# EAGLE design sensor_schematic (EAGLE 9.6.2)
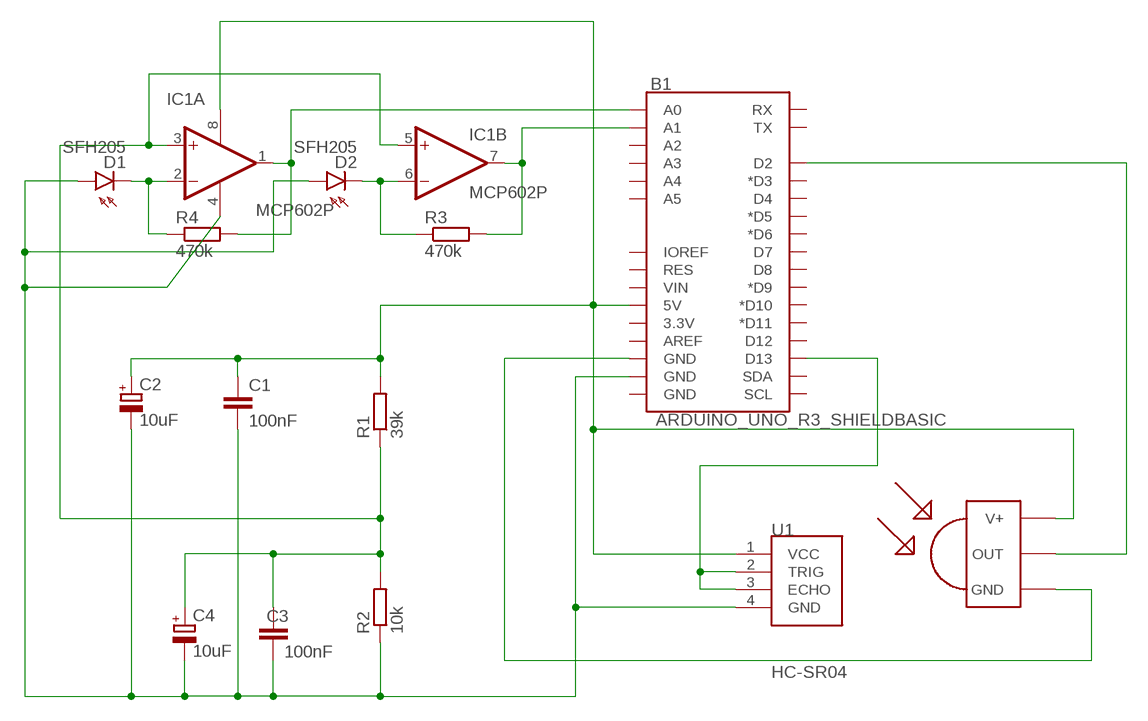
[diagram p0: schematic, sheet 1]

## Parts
B1  ARDUINO_UNO_R3_SHIELDBASIC  [UNO_R3_SHIELD]
C1  100nF  C-EU025-025X050  [C025-025X050]
C2  10uF  CPOL-EUE2.5-6  [E2,5-6]
C3  100nF  C-EU025-025X050  [C025-025X050]
C4  10uF  CPOL-EUE2.5-6  [E2,5-6]
D1  SFH205  [SFH205]
D2  SFH205  [SFH205]
IC1  MCP602P  [DIL08]
R1  39k  R-EU_0207/10  [0207/10]
R2  10k  R-EU_0207/10  [0207/10]
R3  470k  R-EU_0207/10  [0207/10]
R4  470k  R-EU_0207/10  [0207/10]
U1  HC-SR04  [XCVR_HC-SR04]
U$1  TSOP4856  [TSOP18XX]

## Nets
N$2: C3.1 C4.+ IC1.3(A:+IN) IC1.5(B:+IN) R1.1 R2.2
N$3: B1.5V C1.1 C2.+ IC1.8(P:V+) R1.2 U1.1(VCC) U$1.VCC(V+)
N$4: D2.K(C) IC1.6(B:-IN) R3.1
N$5: D1.K(C) IC1.2(A:-IN) R4.1
N$7: B1.GND@1(GND) C1.2 C2.- C3.2 C4.- D1.A D2.A IC1.4(P:V-) R2.1 U1.4(GND)
N$8: B1.GND@2(GND) U$1.GND
N$9: B1.D13 U1.2(TRIG) U1.3(ECHO)
N$10: B1.D2 U$1.OUT
N$11: B1.A0 IC1.1(A:OUT) R4.2
N$12: B1.A1 IC1.7(B:OUT) R3.2
Unconnected: B1.3.3V B1.A2 B1.A3 B1.A4 B1.A5 B1.AREF B1.D3(*D3) B1.D4 B1.D5(*D5) B1.D6(*D6) B1.D7 B1.D8 B1.D9(*D9) B1.D10(*D10) B1.D11(*D11) B1.D12 B1.GND@0(GND) B1.IOREF B1.RES B1.RX B1.SCL B1.SDA B1.TX B1.VIN

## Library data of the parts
B1 = SparkFun-Boards:ARDUINO_UNO_R3_SHIELD: Arduino R3 Shield Footprint Shield form compatible with the Arduino Uno R3. SparkFun Products: MG2639 Cellular Shield MIDI Shield R3 Stackable Headers Kit
C1 C3 = rcl:C-EU: CAPACITOR, European symbol; SPICEPREFIX: C
C2 C4 = rcl:CPOL-EU: POLARIZED CAPACITOR, European symbol; SPICEPREFIX: C
D1 D2 = opto-trans-siemens:SFH205: PHOTO DIODE; OC_FARNELL: unknown; OC_NEWARK: unknown
IC1 = linear:MCP602: Single Op Amp 2.7V to 6.0V Single Supply CMOS Source: http://ww1.microchip.com/downloads/en/DeviceDoc/21314g.pdf
R1-R4 = rcl:R-EU_: RESISTOR, European symbol; SPICEPREFIX: R
U1 = HC-SR04:HC-SR04: Ultrasonic Sensor Module Check availability; AVAILABILITY: Not in stock; DESCRIPTION: HC-SR04 Ultrasonic Sensor Qwiic Platform Evaluation Expansion Board; MF: SparkFun Electronics; MP: HC-SR04; PACKAGE: None; PRICE: None
U$1 = tsop:TSOP4856: IR Receiver and Demodulator

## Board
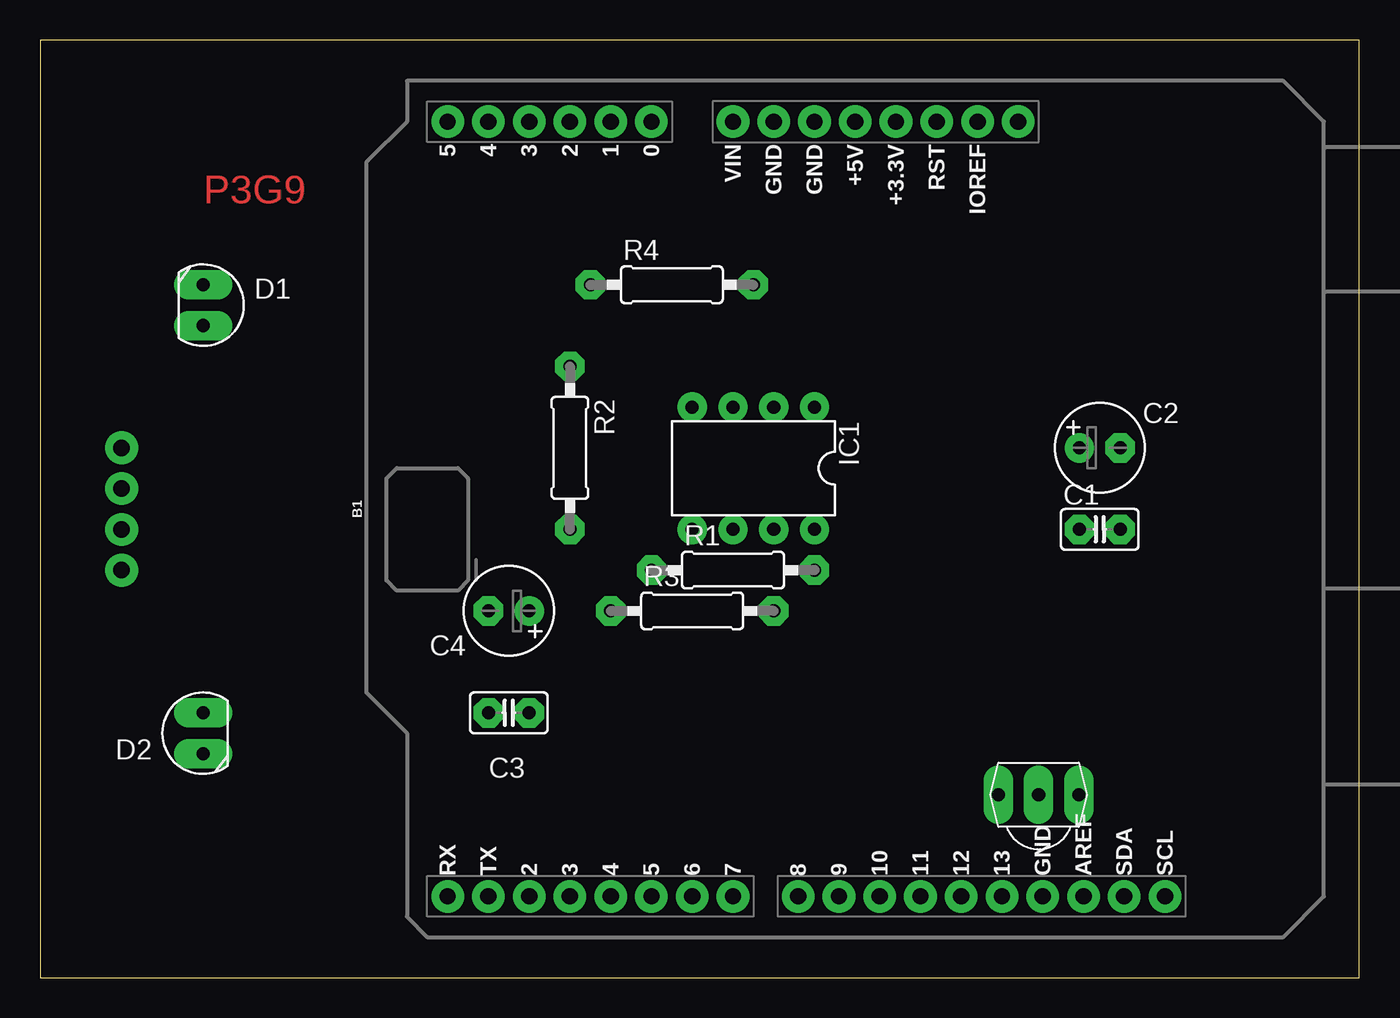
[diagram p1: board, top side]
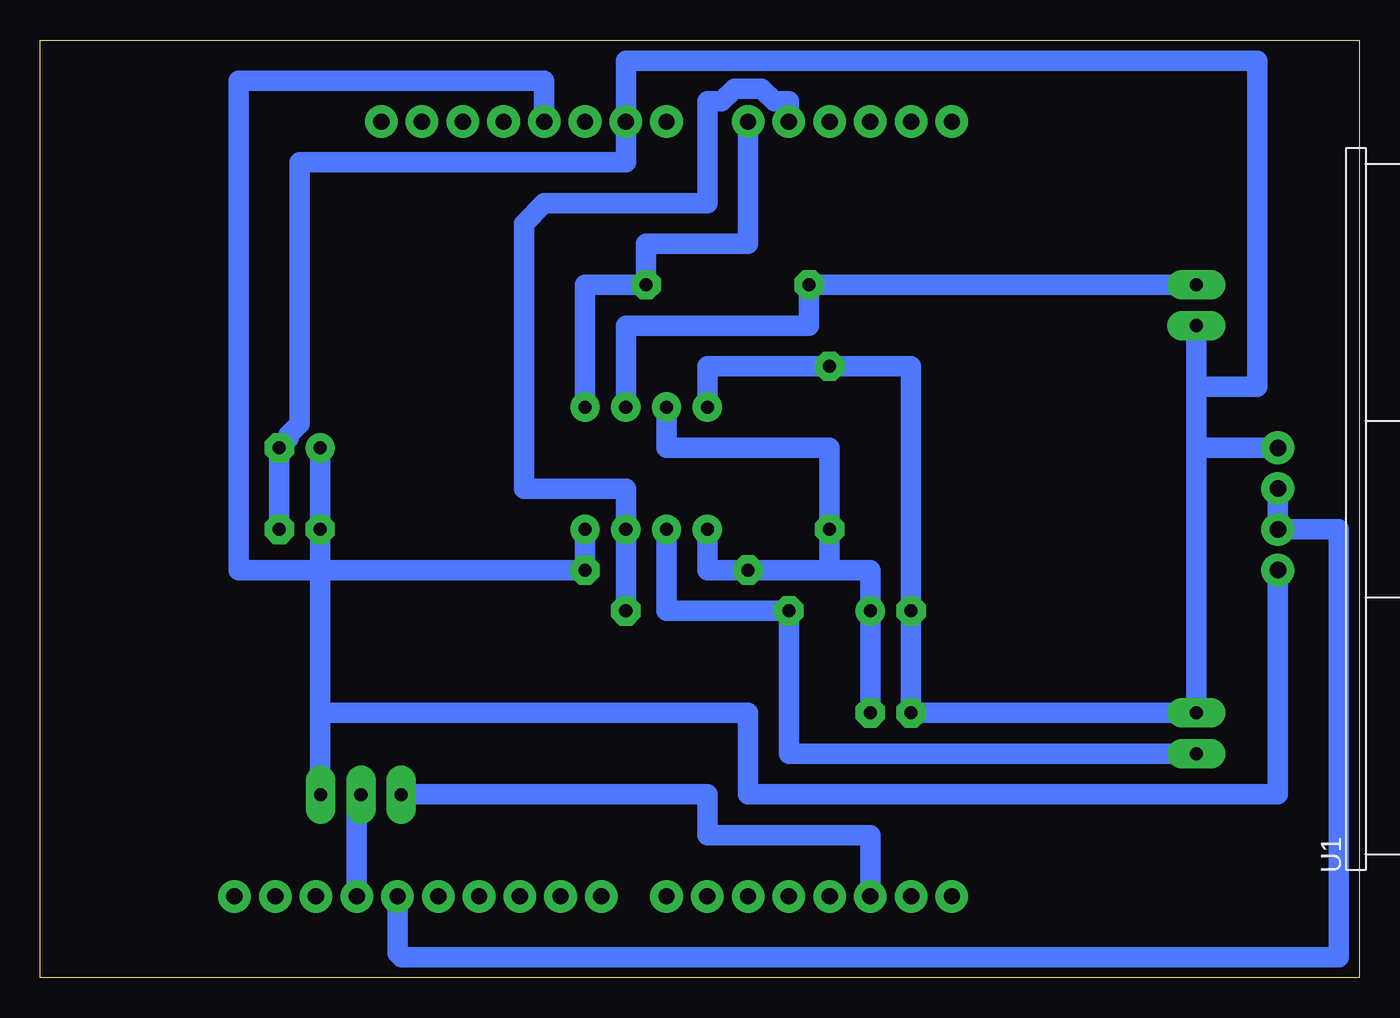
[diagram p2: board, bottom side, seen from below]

Size 82.22 x 58.41 mm. Coordinates in mm from the lower left corner, seen from the top.
Outline: 0,0 82.22,0 82.22,58.41 0,58.41 0,0
Copper layers (1*16): Top 0.035mm / dielectric 1.5mm / Bottom 0.035mm
Design rules "LabE": minimum track width 50mil, minimum drill 0.8mm, track to track 16mil, track to pad 16mil, pad to pad 16mil, via to via 16mil, smd to smd 16mil, copper to edge 0mil, drill to drill 16mil, minimum pad ring 20mil, minimum via ring 20mil, stop-mask expansion 4mil, vias tented up to drill 0mil, thermal gap 10mil

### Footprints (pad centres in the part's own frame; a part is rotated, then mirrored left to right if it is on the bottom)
UNO_R3_SHIELD = drill 1.016 pad 1.88: 3.3V 24.13,-2.54; 5V 24.13,0; A0 24.13,12.7; A1 24.13,15.24; A2 24.13,17.78; A3 24.13,20.32; A4 24.13,22.86; A5 24.13,25.4; AREF -24.13,-14.224; D2 -24.13,20.32; D3 -24.13,17.78; D4 -24.13,15.24; D5 -24.13,12.7; D6 -24.13,10.16; D7 -24.13,7.62; D8 -24.13,3.556; D9 -24.13,1.016; D10 -24.13,-1.524; D11 -24.13,-4.064; D12 -24.13,-6.604; D13 -24.13,-9.144; GND@0 24.13,2.54; GND@1 24.13,5.08; GND@2 -24.13,-11.684; IOREF 24.13,-7.62; NC 24.13,-10.16; RES 24.13,-5.08; RX -24.13,25.4; SCL -24.13,-19.304; SDA -24.13,-16.764; TX -24.13,22.86; VIN 24.13,7.62
C025-025X050 = drill 0.813 octagon: 1 -1.27,0; 2 1.27,0
E2,5-6 = drill 0.813 pad 1.6: + -1.27,0 | drill 0.813 pad 1.6 octagon: - 1.27,0
SFH205 = drill 0.813 long: A 0,-1.27; K 0,1.27
DIL08 = drill 0.813 pad 1.27: 1 -3.81,-3.81; 2 -1.27,-3.81; 3 1.27,-3.81; 4 3.81,-3.81; 5 3.81,3.81; 6 1.27,3.81; 7 -1.27,3.81; 8 -3.81,3.81
0207/10 = drill 0.813 octagon: 1 -5.08,0; 2 5.08,0
XCVR_HC-SR04 = drill 1.02: 1 -3.81,0; 2 -1.27,0; 3 1.27,0; 4 3.81,0
TSOP18XX = drill 0.813 long: GND -0.001,-0.027; OUT -2.501,-0.027; VCC 2.499,-0.027

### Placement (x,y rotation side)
B1  50.8,29.21 90 top
C1  66.04,27.94 0 top
C2  66.04,33.02 0 top
C3  29.21,16.51 180 top
C4  29.21,22.86 180 top
D1  10.16,41.91 0 top
D2  10.16,15.24 180 top
IC1  44.45,31.75 180 top
R1  43.18,25.4 0 top
R2  33.02,33.02 270 top
R3  40.64,22.86 0 top
R4  39.37,43.18 0 top
U1  5.08,29.21 90 bottom
U$1  62.23,11.43 0 top

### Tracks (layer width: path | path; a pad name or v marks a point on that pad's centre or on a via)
N$2
  Bottom 1.27: C3.1 C4.+ 30.48,25.4 33.02,25.4 | 33.02,25.4 R1.1 40.64,25.4 IC1.5 | 33.02,25.4 R2.2 33.02,33.02 43.18,33.02 IC1.3
N$3
  Bottom 1.27: U1.1 5.08,11.43 38.1,11.43 38.1,16.51 64.77,16.51 | 64.77,16.51 64.77,11.45 U$1.VCC | 64.77,25.4 R1.2 IC1.8 | 64.77,25.4 64.77,16.51 | 64.77,25.4 C1.1 C2.+ | 64.77,25.4 69.85,25.4 69.85,55.88 50.8,55.88 B1.5V
N$4
  Bottom 1.27: D2.K 35.56,13.97 R3.1 43.18,22.86 IC1.6
N$5
  Bottom 1.27: D1.K R4.1 34.29,40.64 45.72,40.64 IC1.2
N$7
  Bottom 1.27: D1.A 10.16,36.83 | 10.16,36.83 10.16,33.02 | 10.16,33.02 D2.A C3.2 C4.- 27.94,38.1 R2.1 40.64,38.1 IC1.4 | U1.4 10.16,33.02 | C1.2 C2.- 66.73,33.6 66.73,33.83 66.04,34.52 66.04,50.8 45.72,50.8 B1.GND@1 45.72,57.15 6.35,57.15 6.35,36.83 10.16,36.83
N$8
  Bottom 1.27: U$1.GND 62.48,11.15 B1.GND@2
N$9
  Bottom 1.27: U1.3 U1.2 1.27,27.94 1.27,1.27 59.69,1.27 59.94,1.52 B1.D13
N$10
  Bottom 1.27: B1.D2 30.48,8.89 40.64,8.89 40.64,11.43 59.7,11.43 U$1.OUT
N$11
  Bottom 1.27: IC1.1 48.26,43.18 R4.2 44.45,45.72 38.1,45.72 B1.A0
N$12
  Bottom 1.27: R3.2 IC1.7 45.72,30.48 52.07,30.48 52.07,46.99 50.8,48.26 40.64,48.26 40.64,54.61 39.74,54.61 38.95,55.4 37.25,55.4 36.46,54.61 35.56,54.61 B1.A1

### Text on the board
Top: P3G9

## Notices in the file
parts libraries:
SparkFun-Boards: Licensing: Creative Commons ShareAlike 4.0 International - https://creativecommons.org/licenses/by-sa/4.0
